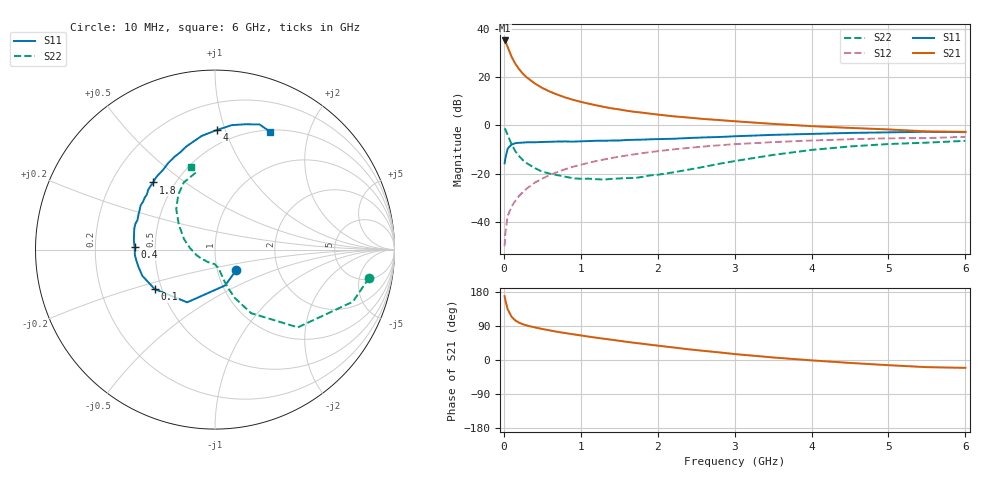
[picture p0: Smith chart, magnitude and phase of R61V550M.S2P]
! SIEMENS Small Signal Semiconductors
! BFR193
! Si NPN RF Bipolar Junction Transistor in SOT23
! VCE = 1.5 V  IC = 50 mA
! Common Emitter S-Parameters:  May  1996
# GHz  S  MA  R  50
!  f  S11  S21  S12  S22
! GHz  MAG  ANG  MAG  ANG  MAG  ANG  MAG  ANG
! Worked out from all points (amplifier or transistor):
!   36 points, 10 MHz to 6 GHz, reference 50 ohm
!   highest |S21| = 35.1 dB at 10 MHz (marker M1)
!   |S21| within 3 dB of that: start of sweep to 53.79 MHz
!   unconditionally stable (mu >= 1): 303.2 MHz to 2.087 GHz
!   at 250 MHz: K = 0.98, MSG = 24.4 dB, |S12| = -27.5 dB
!   at 1.4 GHz: K = 1.03, MAG = 9.2 dB, |S12| = -13.5 dB
!   at 6 GHz: K = 0.98, MSG = 1.0 dB, |S12| = -4.7 dB
!   S11 on the Smith chart (normalised r, x): 10 MHz: 1.23, -0.29; 100 MHz: 0.46, -0.24; 400 MHz: 0.38, +0.01; 1.8 GHz: 0.38, +0.38; 4 GHz: 0.39, +0.94; 6 GHz: 0.52, +1.44
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0.01  0.1645 -43.5  56.89 168.5  0.0032 82.7  0.8734 -10.3
0.02  0.2075 -74.2  54.29 157.6  0.0059 76.8  0.8213 -20.7
0.05  0.3321 -117.8  41.7 133.9  0.0134 68.5  0.6329 -43.2
0.1  0.4018 -146.8  26.4 114.3  0.0211 69.2  0.4073 -60.4
0.15  0.4302 -160.1  18.7 104.2  0.0277 70.0  0.2925 -67.6
0.2  0.437 -167.1  14.4 98.3  0.0351 71.7  0.2303 -70.9
0.25  0.4424 -172.1  11.61 94.1  0.0423 73.0  0.1896 -73.2
0.3  0.4473 -176.1  9.755 91.0  0.05 73.6  0.1651 -74.3
0.4  0.4482 178.0  7.404 86.2  0.0653 74.1  0.132 -76.4
0.5  0.4547 173.7  5.945 81.8  0.0795 73.8  0.1106 -78.6
0.6  0.4589 169.4  4.979 78.0  0.095 73.2  0.1005 -80.8
0.7  0.4646 165.5  4.301 74.2  0.1092 72.1  0.0935 -84.0
0.9  0.4623 159.1  3.385 67.9  0.1399 69.6  0.0807 -91.0
1.1  0.4746 152.2  2.817 61.8  0.169 66.9  0.0794 -100.0
1.4  0.4872 143.2  2.254 53.5  0.2117 62.2  0.0785 -115.2
1.8  0.5083 132.6  1.834 43.0  0.2668 55.8  0.0863 -138.6
2.2  0.5296 123.3  1.545 33.2  0.3192 49.4  0.1071 -163.0
3.5  0.6381 96.6  1.074 6.7  0.452 27.9  0.2456 145.2
4  0.6673 88.9  0.966 -1.0  0.4872 20.8  0.3114 133.9
4.5  0.6998 82.3  0.888 -7.7  0.518 13.7  0.3675 123.9
5.5  0.7401 70.4  0.75 -18.9  0.5479 0.1  0.4404 104.5
6  0.7252 65.1  0.737 -20.7  0.5802 -4.0  0.4796 105.9
